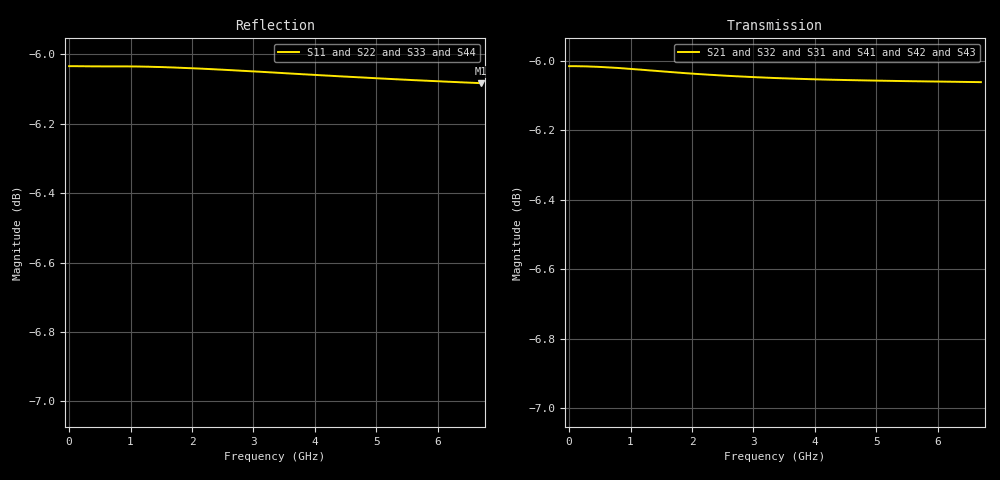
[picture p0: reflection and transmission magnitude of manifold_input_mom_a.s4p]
! Created Mon Jan 20 16:19:32 2014
# ghz S ma R 50
! 4 Port Network Data from data block
! freq  magS11  angS11  magS12  angS12  magS13  angS13  magS14  angS14
!  magS21  angS21  magS22  angS22  magS23  angS23  magS24  angS24
!  magS31  angS31  magS32  angS32  magS33  angS33  magS34  angS34
!  magS41  angS41  magS42  angS42  magS43  angS43  magS44  angS44
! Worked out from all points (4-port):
!   43 points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, 9.306 Hz to 6.7 GHz, reference 50 ohm
!   strongest paths, dB at 9.306 Hz, 372.2 MHz, 1.396 GHz, 3.908 GHz, 6.7 GHz:
!     S21: -6.0, -6.0, -6.0, -6.1, -6.1
!     S32: -6.0, -6.0, -6.0, -6.0, -6.1
!     S31: -6.0, -6.0, -6.0, -6.0, -6.1
!     S41: -6.0, -6.0, -6.0, -6.0, -6.1
!     S42: -6.0, -6.0, -6.0, -6.0, -6.1
!     S43: -6.1, -6.1, -6.2, -6.3, -6.4
!   lowest |S11| = -6.1 dB at 6.7 GHz (marker M1), VSWR 2.97, Z = 16.8 - j0.687 ohm
!   |S11| at or under -10 dB: nowhere
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9.305556e-09  0.4992 -180.0  0.5003 -0.0  0.4994 -0.0  0.4994 -0.0
              0.5003 -0.0  0.4994 -180.0  0.4995 -0.0  0.4995 -0.0
              0.4994 -0.0  0.4995 -0.0  0.4972 -180.0  0.4982 -0.0
              0.4994 -0.0  0.4995 -0.0  0.4982 -0.0  0.4972 -180.0
0.09305556  0.4992 -180.0  0.5003 -0.1  0.4994 -0.1  0.4994 -0.1
            0.5003 -0.1  0.4994 -180.0  0.4995 -0.1  0.4995 -0.1
            0.4994 -0.1  0.4995 -0.1  0.4962 179.8  0.4981 -0.3
            0.4994 -0.1  0.4995 -0.1  0.4981 -0.3  0.4962 179.8
0.4652778  0.4992 -179.9  0.5002 -0.4  0.4996 -0.5  0.4996 -0.5
           0.5002 -0.4  0.4993 -179.8  0.4995 -0.5  0.4994 -0.5
           0.4996 -0.5  0.4995 -0.5  0.4955 179.2  0.4968 -1.4
           0.4996 -0.5  0.4994 -0.5  0.4968 -1.4  0.4955 179.2
0.9305556  0.4992 -179.8  0.4999 -0.7  0.4998 -1.1  0.4998 -1.1
           0.4999 -0.7  0.499 -179.6  0.4995 -1.0  0.4994 -1.0
           0.4998 -1.1  0.4995 -1.0  0.4941 178.4  0.4946 -2.6
           0.4998 -1.1  0.4994 -1.0  0.4946 -2.6  0.4941 178.4
2.233333  0.4988 -179.5  0.4989 -1.6  0.4999 -2.7  0.4999 -2.7
          0.4989 -1.6  0.4989 -179.0  0.4995 -2.4  0.4995 -2.4
          0.4999 -2.7  0.4995 -2.4  0.49 176.7  0.4893 -5.5
          0.4999 -2.7  0.4995 -2.4  0.4893 -5.5  0.49 176.7
4.1875  0.4977 -179.0  0.4981 -2.9  0.499 -5.0  0.4989 -5.0
        0.4981 -2.9  0.4993 -178.0  0.4986 -4.4  0.4986 -4.4
        0.499 -5.0  0.4986 -4.4  0.485 174.5  0.4836 -9.5
        0.4989 -5.0  0.4986 -4.4  0.4836 -9.5  0.485 174.5
6.7  0.4964 -178.2  0.4977 -4.4  0.4972 -7.9  0.4971 -8.0
     0.4977 -4.4  0.5004 -176.9  0.4967 -7.0  0.4967 -7.0
     0.4972 -7.9  0.4967 -7.0  0.4802 171.8  0.4778 -14.5
     0.4971 -8.0  0.4967 -7.0  0.4778 -14.5  0.4802 171.8
